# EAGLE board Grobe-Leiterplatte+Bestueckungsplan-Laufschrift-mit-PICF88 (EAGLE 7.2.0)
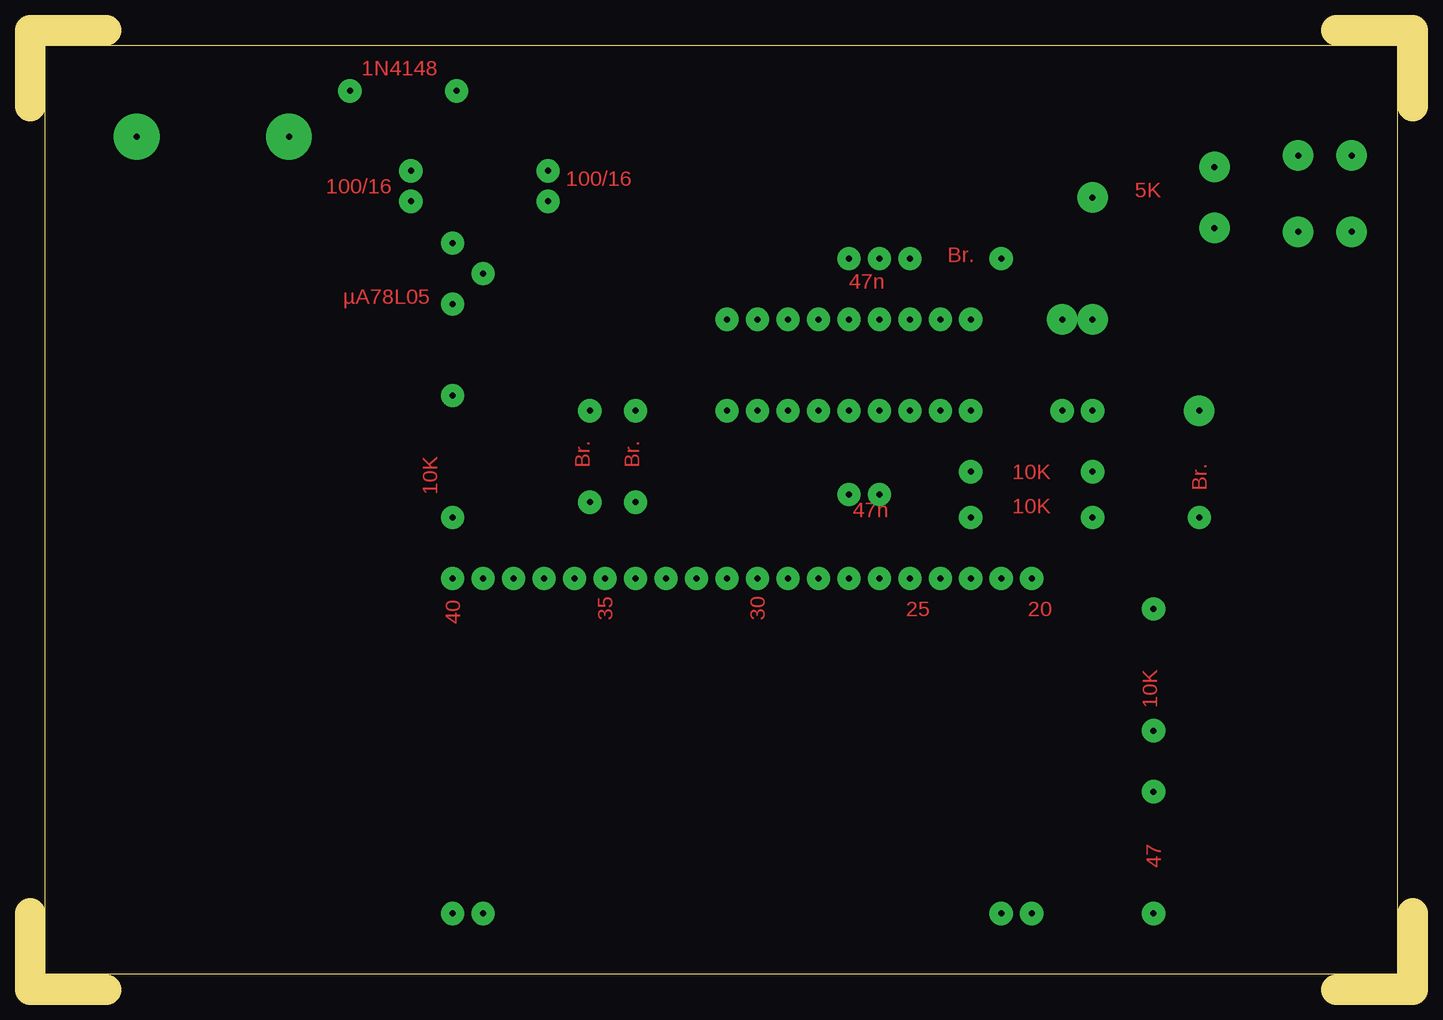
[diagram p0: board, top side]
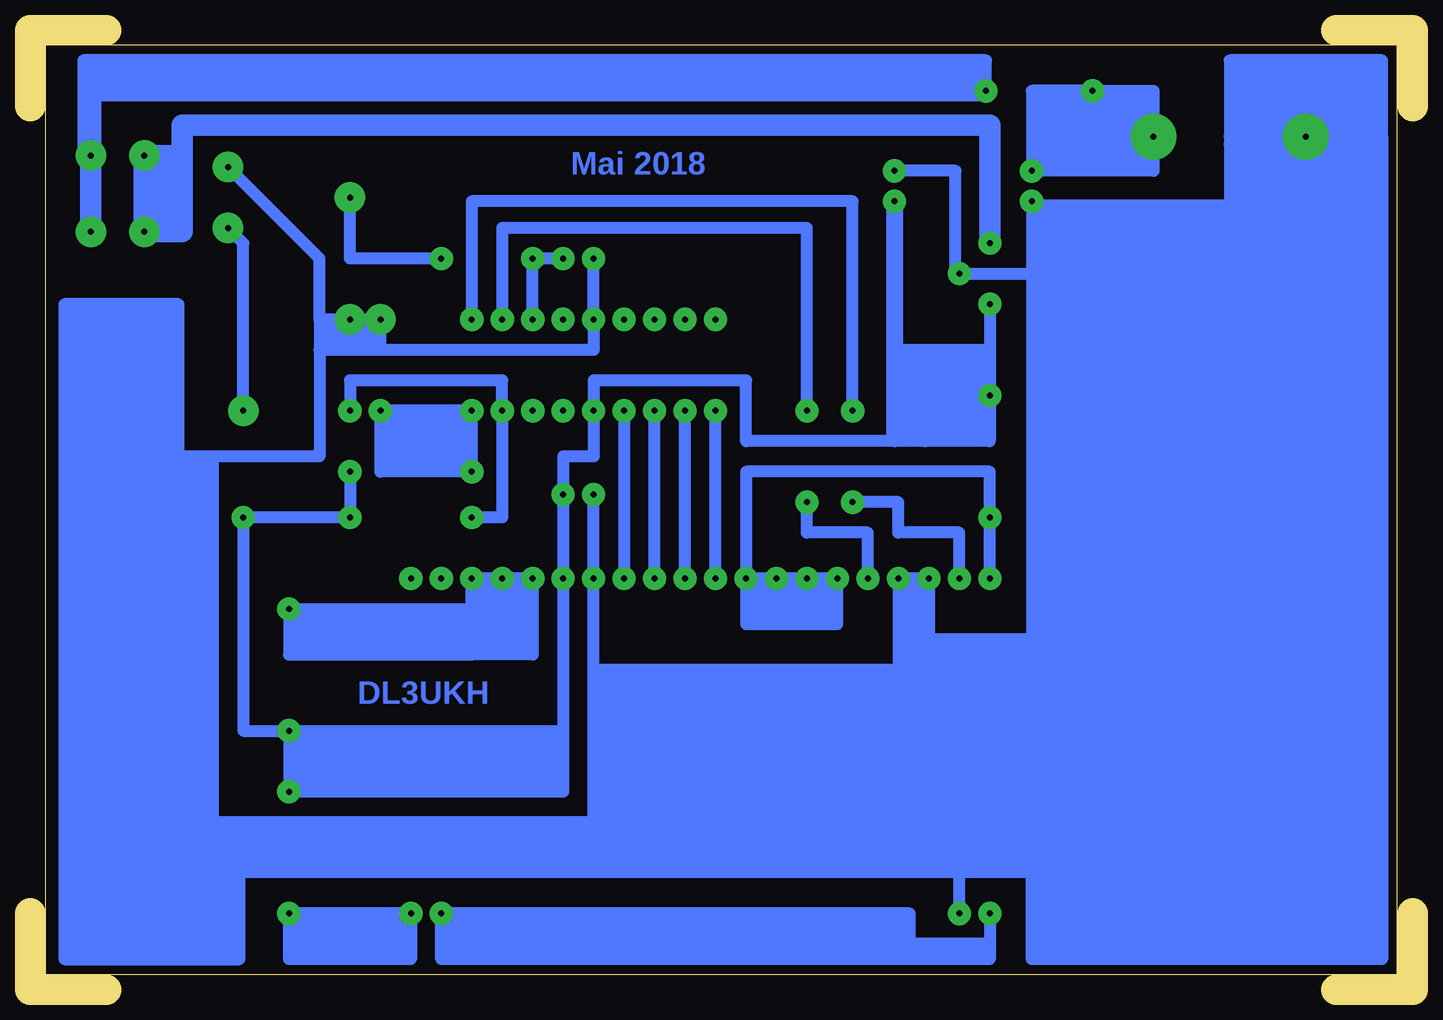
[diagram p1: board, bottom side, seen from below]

Size 115.25 x 80.01 mm. Coordinates in mm from the lower left corner, seen from the top.
Outline: 115.25,73.66 115.25,80.01 108.9,80.01
Outline: 115.25,6.35 115.25,0 108.9,0
Outline: 6.35,0 0,0 0,6.35
Outline: 0,73.66 0,80.01 6.35,80.01
Outline: 113.98,78.74 113.98,1.27 1.27,1.27 1.27,78.74 113.98,78.74
Copper layers (1*16): Top 0.035mm / dielectric 1.5mm / Bottom 0.035mm
Design rules "default": minimum track width 10mil, minimum drill 24mil, track to track 8mil, track to pad 8mil, pad to pad 8mil, via to via 8mil, smd to smd 8mil, copper to edge 40mil, drill to drill 8mil, minimum pad ring 10mil, minimum via ring 8mil, stop-mask expansion 4mil, vias tented up to drill 0mil, thermal gap 10mil

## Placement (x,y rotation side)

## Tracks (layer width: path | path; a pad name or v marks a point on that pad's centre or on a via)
S$1  (via drill 0.5 pad 1.93, 0.5 pad 2.54, 0.5 pad 3.81)
  Bottom 1.016: 99.69,44.45 102.87,44.45 102.87,57.15 112.39,57.15 112.39,9.84 | 112.39,9.84 31.43,9.84 31.43,9.53 | 112.39,9.84 112.39,2.54 97.79,2.54 97.79,10.16 | v37.78,59.69 31.75,59.69 | 31.75,59.69 31.75,29.21 | 86.04,53.34 68.26,53.34 v68.26,55.88 v68.26,60.96 | 91.12,55.88 v88.58,55.88 v86.04,55.88 86.04,53.34 | 91.12,55.88 91.12,53.34 | 91.12,53.34 91.12,44.45 100.01,44.45 100.01,13.97 | v37.78,6.35 37.78,16.51 | 37.78,16.51 40.32,16.51 | 40.32,16.51 42.86,16.51 | 42.86,16.51 68.26,16.51 | 68.26,16.51 v68.26,34.29 v68.26,41.28 | 42.86,26.67 v42.86,34.29 v40.32,34.29 40.32,29.21 | 42.86,26.67 42.86,16.51 | 40.32,29.21 40.32,16.51 | 100.01,13.97 68.26,13.97 | 68.26,13.97 68.26,16.51 | 31.75,29.21 40.32,29.21 | 91.12,55.88 91.12,60.96 v98.74,68.58 | v31.75,65.72 31.75,65.41 | 31.75,65.41 31.75,59.69 | v8.89,71.12 8.89,59.69 31.75,59.69 | v8.89,71.12 2.54,71.12 | 2.54,71.12 2.54,2.54 31.75,2.54 31.75,10.16 | 31.75,10.16 31.75,16.51 | 31.75,16.51 31.75,29.21 | v8.89,71.12 15.24,71.12 | 15.24,71.12 15.24,70.48 15.24,65.41 | 15.24,65.41 15.24,58.1 | 31.75,65.41 15.24,65.41 | 31.75,16.51 37.78,16.51 | 42.86,26.67 67.94,26.67 | 68.26,13.97 27.62,13.97 | 31.75,10.16 97.79,10.16 | 97.79,10.16 100.01,10.16 100.01,13.97 | 86.04,53.34 91.12,53.34 | 2.54,71.12 2.54,77.47 15.24,77.47 15.24,71.12
S$2  (via drill 0.5 pad 1.93)
  Bottom 1.016: v35.24,49.53 35.24,45.72 40.64,45.72 | 40.64,45.72 43.18,45.72 | 43.18,45.72 55.56,45.72 55.56,50.8 68.26,50.8 v68.26,48.26 68.26,44.45 70.8,44.45 v70.8,34.29 70.8,16.51 v93.66,16.51 v93.66,21.59 | v88.58,43.18 v88.58,39.37 v97.47,39.37 97.47,21.59 v93.66,21.59 | v35.24,57.15 35.24,53.34 | 35.24,53.34 v35.24,49.53 | 43.18,45.72 43.18,46.04 40.64,53.34 | v35.24,49.53 40.64,49.53 | 40.64,49.53 40.64,53.34 | v93.66,21.59 71.12,21.59 | 40.64,49.53 40.64,45.72 | 35.24,53.34 40.64,53.34 | 40.64,53.34 42.86,53.34
  Bottom 1.422: v43.18,65.72 43.18,46.04
S$3  (via drill 0.5 pad 1.93)
  Bottom 1.016: v35.24,6.35 35.24,3.81 | 35.24,3.81 35.24,2.54 80.96,2.54 80.96,3.81 | 80.96,3.81 v80.96,6.35 41.91,6.35 41.91,3.81 | 35.24,3.81 41.91,3.81 | 41.91,3.81 80.96,3.81
S$4  (via drill 0.5 pad 1.93)
  Bottom 1.016: v83.5,6.35 v93.66,6.35 93.66,2.54 83.5,2.54 v83.5,6.35
S$5  (via drill 0.5 pad 1.93)
  Bottom 1.016: v45.4,34.29 45.4,38.1 50.48,38.1 v50.48,40.64
S$6  (via drill 0.5 pad 1.93)
  other vias: 70.8,41.28
S$7  (via drill 0.5 pad 1.93, 0.5 pad 3.81)
  Bottom 1.016: v21.59,71.12 21.59,74.93 v26.67,74.93 31.75,74.93 v31.75,68.26 21.59,68.26 21.59,70.8
S$8  (via drill 0.5 pad 1.93)
  Bottom 1.016: 38.1,59.69 38.1,68.26 v43.18,68.26
S$9  (via drill 0.5 pad 1.93, 0.5 pad 2.54)
  Bottom 1.016: v80.96,60.96 88.58,60.96 v88.58,66.04
S$11  (via drill 0.5 pad 1.93)
  Bottom 1.016: v73.34,55.88 v73.34,60.96 v70.8,60.96
S$12  (via drill 0.5 pad 1.93)
  Bottom 1.016: v65.72,48.26 v65.72,34.29
S$13  (via drill 0.5 pad 2.54)
  other vias: 97.47,48.26
S$14  (via drill 0.5 pad 1.93)
  Bottom 1.016: v35.24,34.29 v35.24,39.37 35.24,43.18 55.56,43.18 v55.56,34.29 | v55.56,34.29 55.56,30.48 53.02,30.48 | 53.02,30.48 50.48,30.48 | 50.48,30.48 47.94,30.48 v47.94,34.29 v55.56,34.29 | v50.48,34.29 50.48,30.48 | v53.02,34.29 53.02,30.48
S$15  (via drill 0.5 pad 1.93)
  other vias: 70.8,48.26
S$16  (via drill 0.5 pad 1.93)
  Bottom 1.016: v58.1,34.29 v58.1,48.26
S$17  (via drill 0.5 pad 1.93)
  Bottom 1.016: v60.64,34.29 v60.64,48.26
S$18  (via drill 0.5 pad 1.93)
  Bottom 1.016: v63.18,34.29 v63.18,48.26
S$19  (via drill 0.5 pad 1.93)
  Bottom 1.016: v46.67,48.26 46.67,65.72 78.42,65.72 v78.42,55.88
S$20  (via drill 0.5 pad 1.93)
  other vias: 73.34,48.26
S$21  (via drill 0.5 pad 1.93)
  Bottom 1.016: v75.88,48.26 75.88,39.37 v78.42,39.37
S$22  (via drill 0.5 pad 1.93)
  Bottom 1.016: v78.42,48.26 v78.42,43.18 86.04,43.18 v86.04,48.26 v78.42,48.26
S$23  (via drill 0.5 pad 1.93, 0.5 pad 2.54)
  Bottom 1.778: 102.55,69.53 102.55,63.18 v105.73,63.18 v105.73,69.53 102.55,69.53 | 102.55,69.53 102.55,72.07 35.24,72.07 v35.24,62.23
S$25  (via drill 0.5 pad 1.93)
  other vias: 80.96,34.29
S$26  (via drill 0.5 pad 1.93)
  other vias: 83.5,34.29
S$28  (via drill 0.5 pad 1.93)
  other vias: 70.8,55.88
S$29  (via drill 0.5 pad 1.93)
  Bottom 1.016: 75.88,48.58 75.88,50.8 88.58,50.8 v88.58,48.26
S$30  (via drill 0.5 pad 1.93)
  Bottom 1.016: 78.42,27.94 80.64,27.94 93.66,27.94 v93.66,31.75 78.42,31.75 | 73.34,30.48 v73.34,34.29 v78.42,34.29 78.42,31.75 | 73.34,30.48 75.88,30.48 | 75.88,30.48 v75.88,34.29 | 75.88,30.48 78.42,30.48 | 78.42,30.48 78.42,31.75 | 78.42,27.94 78.42,30.48 | 73.34,30.48 73.34,27.94 78.42,27.94
S$31  (via drill 0.5 pad 2.54)
  Bottom 1.016: 97.47,47.94 97.47,62.23 v98.74,63.5
S$32  (via drill 0.5 pad 1.93)
  other vias: 65.72,55.88
S$33  (via drill 0.5 pad 1.93)
  other vias: 63.18,55.88
S$34  (via drill 0.5 pad 1.93)
  other vias: 60.64,55.88
S$35  (via drill 0.5 pad 1.93)
  other vias: 58.1,55.88
S$37  (via drill 0.5 pad 1.93)
  Bottom 1.016: v50.48,48.26 50.48,63.5 75.88,63.5 v75.88,55.88
S$38  (via drill 0.5 pad 1.93)
  Bottom 1.016: v37.78,34.29 37.78,38.1 42.86,38.1 42.86,40.64 v46.67,40.64
S$40  (via drill 0.5 pad 1.93, 0.5 pad 2.54)
  Bottom 1.016: 110.17,69.21 v110.17,69.53 | v35.56,74.93 35.56,77.47 110.81,77.47 110.81,69.21 110.49,69.21
  Bottom 1.778: v35.56,74.93 110.17,74.93 v110.17,69.53 v110.17,63.18
(copper drawn outside any net)
  shapes: Bottom area x27

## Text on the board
Top: 1N4148 | 100/16 | 100/16 | 5K | Br. | µA78L05 | 47n | 10K | Br. | Br. | 10K | 10K | Br. | 47n | 35 | 30 | 25 | 20 | 40 | 10K | 47
Bottom: Mai 2018 | DL3UKH
Pads: AUF BESTÜCKUNGS-SEITE GESEHEN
